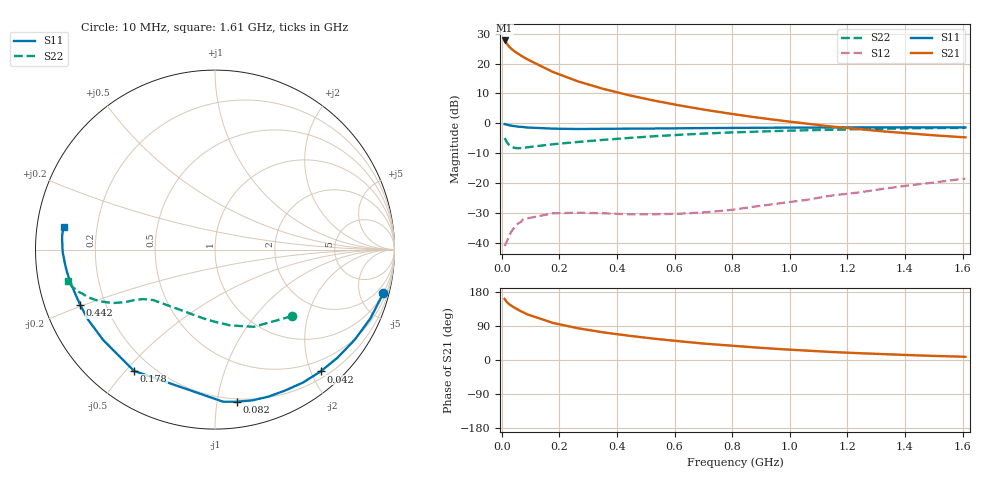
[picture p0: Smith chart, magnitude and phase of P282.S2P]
# MHZ S MA R 50
! Date: Thu Jul 13 17:08:27 1995
!  POLYFET RF DEVICES
!  P282
!  S PARAMETERS
!  VDS=28V, IDQ=1.20mA
!  FREQ  S11MAG  S11ANG  S21MAG  S21ANG  S12MAG  S12ANG  S22MAG  S22ANG
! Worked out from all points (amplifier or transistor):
!   29 points, 10 MHz to 1.61 GHz, reference 50 ohm
!   highest |S21| = 27.8 dB at 10 MHz (marker M1)
!   |S21| within 3 dB of that: start of sweep to 36.05 MHz
!   unconditionally stable (mu >= 1): 450 MHz to 1.005 GHz
!   at 42 MHz: K = 0.11, MSG = 29.8 dB, |S12| = -35.2 dB
!   at 442 MHz: K = 0.99, MSG = 20.0 dB, |S12| = -30.5 dB
!   at 1.61 GHz: K = 0.38, MSG = 6.9 dB, |S12| = -18.6 dB
!   S11 on the Smith chart (normalised r, x): 10 MHz: 0.98, -7.76; 42 MHz: 0.31, -2.15; 82 MHz: 0.18, -1.14; 178 MHz: 0.13, -0.53; 442 MHz: 0.11, -0.20; 1.61 GHz: 0.08, +0.07
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10  0.969 -14.5  24.47 161.2  0.00869 65.9  0.5653 -41.0
18  0.947 -23.9  21.46 152.6  0.01047 58.9  0.4816 -63.3
26  0.9267 -32.8  19.22 147.2  0.01309 55.3  0.4307 -78.6
34  0.9103 -41.4  17.64 143.0  0.01537 53.5  0.4025 -89.9
42  0.8984 -49.1  16.43 139.2  0.01736 48.5  0.3896 -98.5
50  0.8883 -56.4  15.4 135.6  0.01961 48.4  0.3835 -105.5
58  0.877 -63.6  14.54 132.2  0.021 45.8  0.3823 -110.9
66  0.8715 -70.1  13.74 129.0  0.0221 42.7  0.3835 -115.5
74  0.8654 -76.0  13.01 125.9  0.02437 40.8  0.3868 -119.3
82  0.8564 -81.8  12.35 123.0  0.02527 37.5  0.391 -122.5
90  0.8487 -86.9  11.75 120.2  0.02549 37.4  0.396 -125.3
178  0.8127 -123.7  7.241 97.8  0.0309 24.8  0.4451 -140.8
266  0.8013 -141.2  5.017 83.6  0.03164 21.1  0.4869 -145.5
354  0.8082 -151.4  3.758 72.8  0.0309 21.5  0.5276 -147.9
442  0.8118 -157.7  2.951 64.0  0.02975 25.2  0.5676 -149.3
530  0.8169 -162.6  2.396 56.2  0.02974 31.4  0.6058 -150.9
618  0.8237 -166.4  1.989 49.4  0.03047 37.8  0.6409 -152.3
706  0.8306 -169.7  1.682 43.1  0.0321 45.8  0.6733 -154.2
882  0.8398 -174.7  1.257 33.0  0.04028 59.3  0.7233 -157.2
1146  0.8502 179.4  0.8811 21.1  0.06143 67.5  0.7771 -161.5
1410  0.855 174.6  0.6798 13.1  0.09044 68.3  0.8203 -165.1
1610  0.8523 171.6  0.5816 8.4  0.118 65.4  0.8382 -167.9
